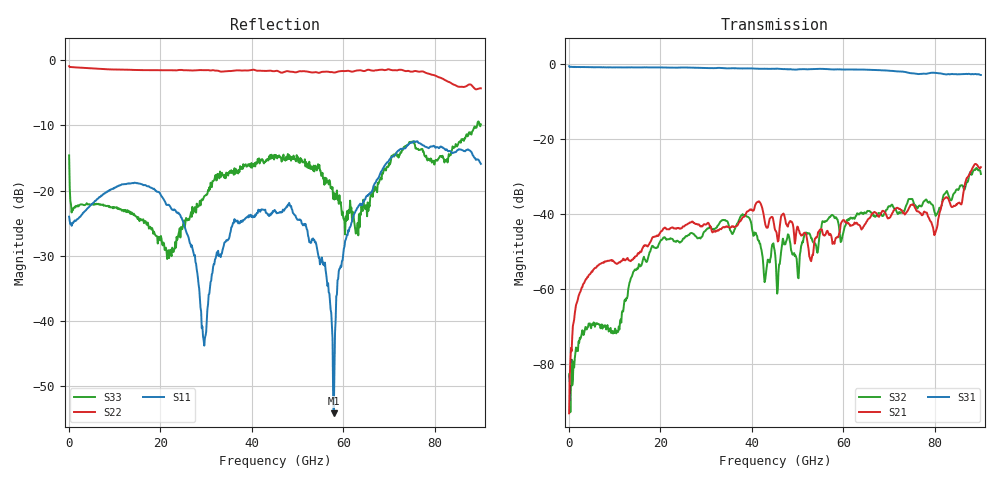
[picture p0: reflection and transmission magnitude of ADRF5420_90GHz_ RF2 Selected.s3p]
! Device:  ADRF5420
! Description: Flip-Chip, Silicon SPDT Switch
! Frequency:  0.1 GHz -  90 GHz
! Ports:
!  RFC = Port 1
!  RF1 = Port 2
!  RF2 = Port 3
! VDD  =  +3.3 Volts
! VSS  =  -3.3 Volts
! State
! RF2 Selected: CTRL = 0 V
! Data:  Data was collected using a calibrated network analyzer
!  The reference plane is the package boundry of ADRF5420 switch.
! Notes: Analog Devices supplies this data as a sample of measured data
!  for this product.  Your particular data for this product may vary.
!  Analog Devices reserves the right to change this data at anytime.
# GHz S  dB  R 50
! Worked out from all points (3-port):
!   656 points, 50 MHz to 90.07 GHz, reference 50 ohm
!   strongest paths, dB at 50 MHz, 22.59 GHz, 45.13 GHz, 67.67 GHz, 90.07 GHz:
!     S31: -0.5, -0.9, -1.2, -1.6, -2.9
!     S21: -93.0, -43.5, -44.3, -40.6, -27.4
!     S32: -82.6, -46.6, -51.1, -39.7, -29.3
!   lowest |S11| = -54.2 dB at 57.91 GHz (marker M1), VSWR 1.00, Z = 49.8 + j0.0825 ohm
!   |S11| at or under -10 dB: start of sweep to end of sweep
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0.05  -24.02 -28.7  -82.61 -172.7  -0.67 0.8
      -93.03 -164.7  -0.91 -178.7  -83.36 125.2
      -0.54 1.3  -82.62 179.7  -14.60 42.5
5.272625  -21.92 8.1  -54.84 62.0  -0.80 -34.5
          -54.90 62.0  -1.27 151.2  -69.10 37.3
          -0.81 -33.9  -69.49 36.8  -22.11 -10.0
15.30556  -18.92 -38.9  -50.48 60.0  -0.86 -99.5
          -50.48 61.3  -1.48 101.8  -53.30 125.2
          -0.88 -97.5  -53.27 125.6  -24.45 -52.3
26.30056  -27.60 -108.7  -42.37 18.8  -0.92 -172.4
          -42.37 21.6  -1.55 51.7  -45.52 22.0
          -0.92 -168.6  -45.51 23.0  -24.52 154.2
29.59906  -43.81 156.5  -42.53 2.5  -1.01 165.7
          -42.62 4.0  -1.52 37.1  -44.68 5.0
          -1.01 169.8  -44.64 7.3  -20.88 121.9
45.1295  -23.23 -26.4  -44.31 -82.8  -1.22 63.2
         -44.30 -79.2  -1.64 -30.5  -51.15 -154.4
         -1.21 68.7  -51.11 -154.0  -14.94 3.2
57.91119  -54.21 154.8  -47.78 -124.9  -1.40 -24.8
          -47.44 -114.9  -1.88 -86.4  -40.39 92.8
          -1.41 -14.4  -40.53 94.1  -20.35 -96.0
62.58406  -23.33 33.2  -42.37 -157.2  -1.34 -57.5
          -42.38 -146.7  -1.63 -108.0  -40.85 58.2
          -1.43 -46.6  -40.88 59.8  -25.88 -83.4
79.07656  -13.22 -104.8  -41.68 111.1  -2.30 -177.1
          -41.91 120.8  -2.16 161.7  -37.18 -56.5
          -2.34 -166.0  -36.98 -55.2  -15.08 -104.4
90.07156  -15.91 124.4  -27.68 102.6  -3.41 91.5
          -27.45 115.0  -4.31 90.7  -29.52 -140.0
          -2.89 103.0  -29.28 -140.5  -9.85 -105.2
